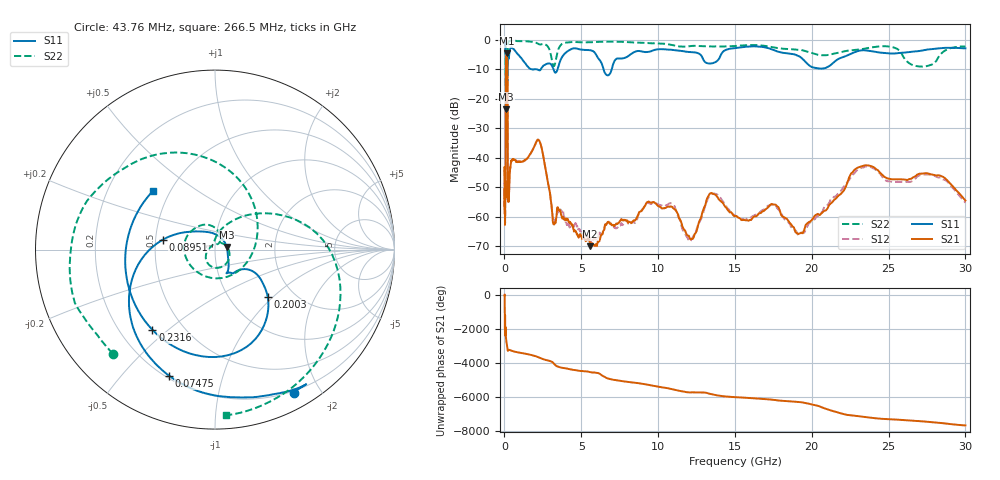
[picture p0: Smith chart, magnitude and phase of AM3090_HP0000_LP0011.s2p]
! Date/Time: Thu, Feb 28, 2019 1:52 PM
! Network Analyzer: Agilent Technologies E8364B Rev: A.07.50.67
! Sweep from 0.010 to 30.000 GHz, 1601 Points, Sweep Type: LOG
! Power Supply: 5.023 V, 0.002 A
# Hz S DB R 50
!freq MagS11 AngS11 MagS21 AngS21 MagS12 AngS12 MagS22 AngS22
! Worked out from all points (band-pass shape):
!   1601 points, 10 MHz to 30 GHz, reference 50 ohm
!   highest |S21| = -4.47 dB at 137 MHz (marker M1); lowest = -70.0 dB at 5.584 GHz (marker M2)
!   |S21| within 3 dB of the highest: 98.35 MHz to 187.7 MHz (89.38 MHz wide, 62.5 % of centre)
!   lowest |S11| = -23.5 dB at 97.94 MHz (marker M3), VSWR 1.14, Z = 56.9 + j1.7 ohm
!   |S11| at or under -10 dB: 2.132 GHz to 2.361 GHz (229.1 MHz wide, 10.2 % of centre); 3.197 GHz to 3.456 GHz (259.3 MHz wide, 7.79 % of centre); 6.455 GHz to 6.98 GHz (525.7 MHz wide, 7.83 % of centre)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
!   |S22| runs from -31.5 to -0.2 dB; largest |S21 - S12| = 0.012
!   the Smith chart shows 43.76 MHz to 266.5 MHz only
!   S11 on the Smith chart (normalised r, x): 43.76 MHz: 0.18, -1.68; 74.75 MHz: 0.21, -0.68; 89.51 MHz: 0.55, +0.07; 200.3 MHz: 1.49, -0.92; 231.6 MHz: 0.34, -0.44; 266.5 MHz: 0.40, +0.34
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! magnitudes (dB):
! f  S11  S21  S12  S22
! 10 MHz  -0.2  -44.7  -44.4  -0.5
! 38.04 MHz  -0.5  -58.5  -60.4  -1.4
! 43.76 MHz  -0.8  -56.8  -61.2  -1.8
! 74.75 MHz  -2.5  -44.4  -44.5  -4.7
! 89.51 MHz  -10.6  -14.8  -14.7  -15.8
! 97.94 MHz  -23.5  -7.6  -7.6  -15.3
! 137 MHz  -16.1  -4.5  -4.5  -24.8
! 144.7 MHz  -15.7  -4.5  -4.5  -21.4
! 179.4 MHz  -14.1  -6.1  -6.1  -31.4
! 200.3 MHz  -8.1  -13.5  -13.5  -12.0
! 231.6 MHz  -4.9  -54.3  -54.2  -1.6
! 266.5 MHz  -6.5  -54.1  -54.2  -0.7
! 550.5 MHz  -2.9  -40.5  -40.8  -0.2
! 2.084 GHz  -10.0  -34.5  -34.4  -1.0
! 3.22 GHz  -10.4  -62.6  -62.3  -8.9
! 5.584 GHz  -3.5  -70.0  -67.6  -0.8
! 7.926 GHz  -5.9  -61.4  -61.2  -0.7
! 12.07 GHz  -4.1  -67.4  -68.5  -2.1
! 13.68 GHz  -7.6  -52.4  -52.1  -2.2
! 19.31 GHz  -6.0  -65.5  -65.4  -3.4
! 23.48 GHz  -3.5  -42.6  -43.0  -2.9
! 30 GHz  -2.8  -54.5  -55.3  -2.2
